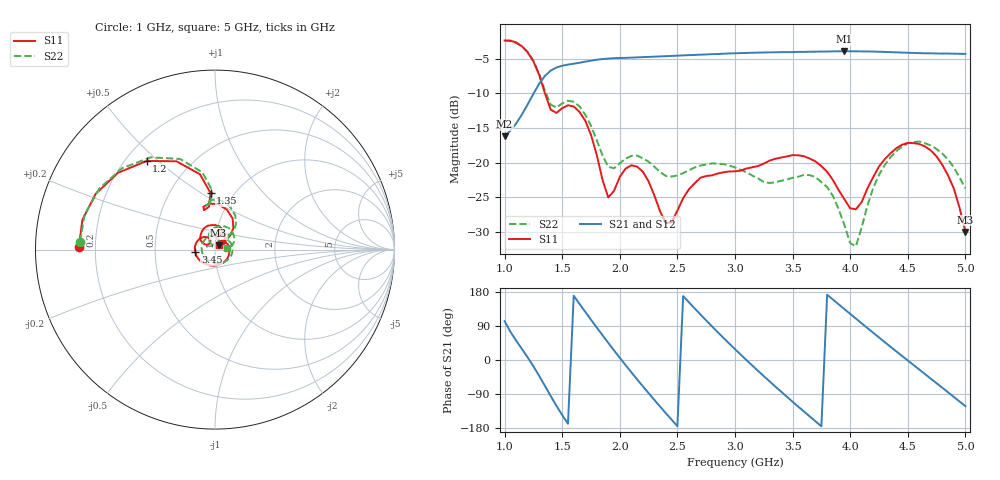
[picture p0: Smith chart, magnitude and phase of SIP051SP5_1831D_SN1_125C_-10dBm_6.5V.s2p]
# GHz  S  dB  R  50
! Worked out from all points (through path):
!   81 points, 1 GHz to 5 GHz, reference 50 ohm
!   highest |S21| = -3.95 dB at 3.95 GHz (marker M1); lowest = -16.2 dB at 1 GHz (marker M2)
!   lowest |S11| = -30.0 dB at 5 GHz (marker M3), VSWR 1.07, Z = 51.9 + j2.57 ohm
!   |S11| at or under -10 dB: 1.35 GHz to end of sweep
!   |S22| runs from -32.1 to -2.5 dB; largest |S21 - S12| = 0.0019
!   S11 on the Smith chart (normalised r, x): 1 GHz: 0.14, +0.01; 1.2 GHz: 0.28, +0.46; 1.35 GHz: 0.78, +0.55; 3.45 GHz: 0.80, -0.02; 5 GHz: 1.04, +0.05
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1  -2.40 178.8  -16.21 102.5  -16.20 102.6  -2.45 176.7
1.2  -4.10 127.6  -11.62 6.9  -11.62 6.8  -4.06 124.8
1.35  -10.01 94.5  -7.51 -68.4  -7.51 -68.4  -9.62 92.8
1.45  -12.84 105.6  -6.30 -120.8  -6.27 -120.8  -12.06 100.8
1.55  -11.74 97.7  -5.88 -168.3  -5.87 -168.3  -11.09 92.3
1.7  -13.97 60.8  -5.45 127.1  -5.45 127.2  -13.10 59.5
1.9  -25.03 63.4  -5.01 45.2  -5.00 45.2  -20.62 54.5
2  -22.06 84.3  -4.92 5.7  -4.91 5.7  -20.11 67.0
2.2  -21.32 46.4  -4.80 -69.4  -4.81 -69.4  -19.39 47.6
2.35  -27.04 31.3  -4.70 -123.0  -4.69 -123.0  -21.36 38.5
2.55  -25.13 55.1  -4.55 168.7  -4.54 168.7  -21.53 38.1
2.75  -21.95 8.1  -4.42 104.3  -4.40 104.3  -20.27 16.8
3  -21.27 -66.5  -4.25 28.6  -4.24 28.6  -20.71 -33.6
3.2  -20.50 -118.6  -4.15 -28.7  -4.15 -28.7  -22.29 -94.2
3.45  -19.12 -172.9  -4.08 -96.8  -4.07 -96.8  -22.45 171.1
3.7  -19.85 139.6  -4.02 -162.1  -4.01 -162.2  -22.12 98.9
3.95  -25.30 117.8  -3.95 134.3  -3.95 134.3  -29.00 64.3
4.05  -26.74 139.3  -3.96 109.2  -3.96 109.2  -32.05 104.4
4.35  -18.67 132.9  -4.08 35.0  -4.09 35.0  -19.25 101.4
4.6  -17.33 88.3  -4.23 -25.3  -4.22 -25.3  -16.97 55.9
4.8  -20.33 54.4  -4.29 -73.4  -4.28 -73.3  -18.71 23.2
5  -30.01 51.4  -4.34 -121.8  -4.35 -121.9  -23.75 7.4
